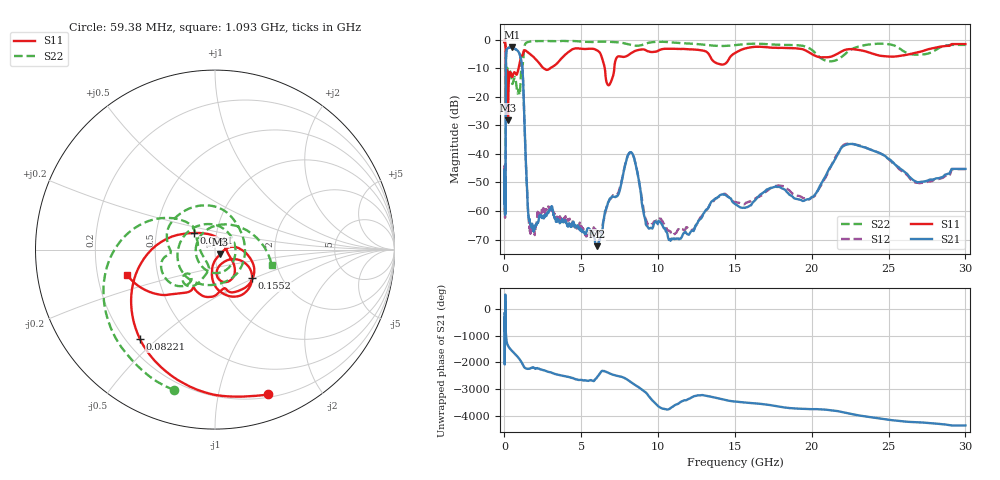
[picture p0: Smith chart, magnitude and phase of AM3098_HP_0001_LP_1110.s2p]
! Date/Time: Thu, Feb 28, 2019 8:32 AM
! Network Analyzer: Agilent Technologies E8364B Rev: A.07.50.67
! Sweep from 0.010 to 30.000 GHz, 1601 Points, Sweep Type: LOG
! Power Supply: 5.023 V, 0.002 A
# Hz S DB R 50
!freq MagS11 AngS11 MagS21 AngS21 MagS12 AngS12 MagS22 AngS22
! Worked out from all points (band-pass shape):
!   1601 points, 10 MHz to 30 GHz, reference 50 ohm
!   highest |S21| = -2.77 dB at 495.6 MHz (marker M1); lowest = -72.3 dB at 6.019 GHz (marker M2)
!   |S21| within 3 dB of the highest: 105.9 MHz to 1.027 GHz (921.5 MHz wide, 163 % of centre)
!   lowest |S11| = -28.3 dB at 232.8 MHz (marker M3), VSWR 1.08, Z = 53 - j2.64 ohm
!   |S11| at or under -10 dB: 91.07 MHz to 922.3 MHz (831.2 MHz wide, 164 % of centre); 2.533 GHz to 2.995 GHz (461.8 MHz wide, 16.7 % of centre); 6.527 GHz to 7.151 GHz (624.2 MHz wide, 9.13 % of centre)
!   |S22| runs from -22.4 to -0.5 dB; largest |S21 - S12| = 0.011
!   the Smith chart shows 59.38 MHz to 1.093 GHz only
!   S11 on the Smith chart (normalised r, x): 59.38 MHz: 0.23, -1.40; 82.21 MHz: 0.26, -0.44; 94.1 MHz: 0.78, +0.15; 155.2 MHz: 1.42, -0.49; 1.093 GHz: 0.33, -0.13
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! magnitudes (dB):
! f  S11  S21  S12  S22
! 10 MHz  -0.3  -46.1  -44.9  -0.6
! 38.04 MHz  -0.5  -60.5  -61.5  -1.0
! 59.38 MHz  -1.3  -51.0  -50.5  -1.8
! 71.82 MHz  -2.0  -51.6  -51.9  -2.5
! 82.21 MHz  -3.7  -33.3  -34.0  -4.2
! 94.1 MHz  -16.5  -11.8  -11.7  -20.3
! 144.7 MHz  -14.5  -3.5  -3.5  -12.7
! 155.2 MHz  -11.7  -3.4  -3.4  -11.0
! 232.8 MHz  -28.3  -2.9  -2.9  -12.0
! 308.1 MHz  -12.5  -2.9  -2.8  -11.2
! 495.6 MHz  -13.1  -2.8  -2.8  -15.3
! 550.5 MHz  -12.5  -3.0  -2.9  -15.1
! 1.093 GHz  -5.9  -7.4  -7.4  -9.7
! 1.598 GHz  -4.8  -63.2  -64.5  -0.8
! 2.084 GHz  -7.1  -64.6  -64.5  -0.5
! 6.019 GHz  -3.8  -72.3  -68.3  -0.8
! 6.821 GHz  -15.9  -56.2  -56.2  -0.8
! 7.926 GHz  -5.9  -42.5  -42.2  -1.5
! 11.08 GHz  -3.3  -69.9  -68.1  -1.1
! 19.8 GHz  -4.4  -55.8  -56.1  -3.0
! 22.67 GHz  -3.4  -36.6  -36.6  -3.2
! 30 GHz  -1.6  -45.3  -45.4  -1.9
